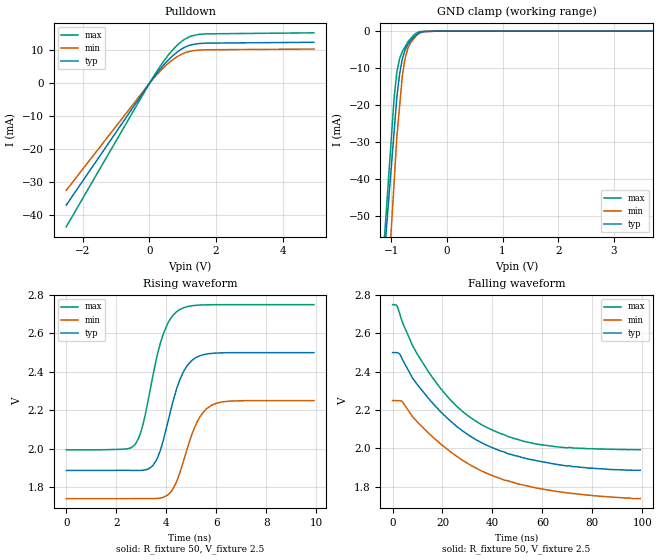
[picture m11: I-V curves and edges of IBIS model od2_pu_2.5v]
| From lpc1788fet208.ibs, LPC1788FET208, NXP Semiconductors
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[Model]   od2_pu_2.5v
Model_type I/O_open_drain
Vinl=7.500E-01
Vinh=1.750E+00
Vref=2.500E+00
Rref=2.000E+03
Cref=0.000E+00
Vmeas=1.250E+00
C_comp   5.160E-13   4.910E-13   5.420E-13
[Voltage Range]   2.500E+00   2.250E+00   2.750E+00
[POWER Clamp Reference]   2.500E+00   2.250E+00   2.750E+00
[GND Clamp Reference]   0.000E+00   0.000E+00   0.000E+00
[Pullup Reference]   2.500E+00   2.250E+00   2.750E+00
[Pulldown Reference]   0.000E+00   0.000E+00   0.000E+00
[Temperature Range]   25   85   -40
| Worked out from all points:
|   slope of the pulldown table from 0 to 0.375 V, typ, clamps not added: 75.7 ohm
|   GND clamp passes 1 mA (typ) near -0.55 V on its own axis
|   rising waveform, R_fixture 50, V_fixture 2.5: 20-80 % time 802ps typ, 818ps min, 783ps max; typ from 1.89 V to 2.5 V
|   falling waveform, R_fixture 50, V_fixture 2.5: 20-80 % time 31.4ns typ, 34.3ns min, 27.2ns max; typ from 2.5 V to 1.89 V
[GND Clamp]
-2.5V     -320.9mA   -428.2mA   -355.8mA
-950mV    -27.31mA   -41.03mA   -18.18mA
-900mV    -17.84mA   -28.54mA   -11.01mA
-850mV    -11.49mA   -20.22mA   -7.415mA
-800mV    -7.413mA   -11.9mA    -5.476mA
-750mV    -5.014mA   -7.253mA   -4.181mA
-700mV    -3.535mA   -4.543mA   -2.887mA
-650mV    -2.594mA   -3.07mA    -2.015mA
-550mV    -1.057mA   -1.212mA   -539.5uA
-400mV    -147.5uA   -112.4uA   -63.11uA
-200mV    -36.9uA    -30.37uA   -38.72uA
5V        16.89uA    16.03uA    16.38uA
[Pulldown]
-2.5V     -37.02mA   -32.52mA   -43.62mA
152.9mV   2.149mA    1.866mA    2.564mA
591.7mV   7.38mA     6.328mA    8.925mA
771.2mV   9.017mA    7.692mA    10.96mA
970.7mV   10.47mA    8.879mA    12.79mA
1.27V     11.72mA    9.839mA    14.4mA
1.629V    12.19mA    10.19mA    15.01mA
4.94V     12.49mA    10.42mA    15.36mA
[Rising Waveform]
R_fixture = 50
V_fixture = 2.5
V_fixture_min = 2.25
V_fixture_max = 2.75
0s        1.887V     1.739V     1.994V
2.376ns   1.887V     1.739V     1.998V
2.772ns   1.886V     1.74V      2.025V
3.069ns   1.887V     1.74V      2.126V
3.6ns     1.939V     1.74V      2.465V
4.059ns   2.137V     1.758V     2.653V
4.555ns   2.363V     1.879V     2.726V
5.148ns   2.471V     2.116V     2.746V
5.8ns     2.496V     2.225V     2.75V
9.901ns   2.5V       2.25V      2.75V
[Falling Waveform]
R_fixture = 50
V_fixture = 2.5
V_fixture_min = 2.25
V_fixture_max = 2.75
0s        2.5V       2.25V      2.75V
1.798ns   2.5V       2.249V     2.743V
3.896ns   2.465V     2.245V     2.66V
8.591ns   2.357V     2.157V     2.523V
17.28ns   2.219V     2.046V     2.346V
25.77ns   2.114V     1.958V     2.219V
35.07ns   2.034V     1.887V     2.128V
46.15ns   1.973V     1.832V     2.063V
58.04ns   1.935V     1.793V     2.022V
99.2ns    1.887V     1.739V     1.994V
[Ramp]
dV/dt_r   3.6807E-01/7.9470E-10   3.0650E-01/8.1600E-10   4.5371E-01/7.7670E-10
dV/dt_f   3.6807E-01/3.1494E-08   3.0650E-01/3.4327E-08   4.5371E-01/2.7399E-08
R_load = 50
